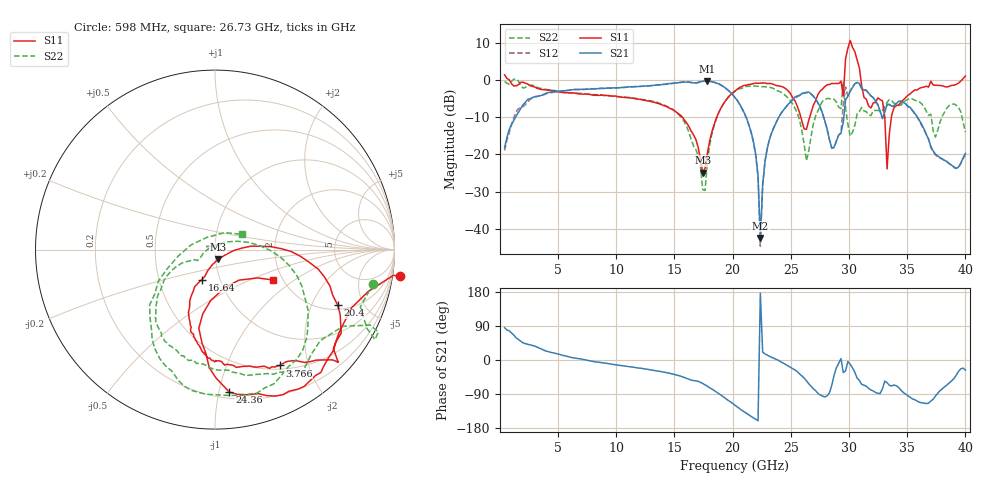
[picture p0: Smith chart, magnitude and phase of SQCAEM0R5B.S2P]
! Network Analyzer HP8722ES.07.66: Jul 25, 2000 Serial No. US39175408
! 26 Oct 2004  08:55:13
! Frequency  S11  S21  S12  S22
# HZ  S  DB R  50
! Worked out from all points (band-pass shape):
!   201 points, 400 MHz to 40 GHz, reference 50 ohm
!   highest |S21| = -0.34 dB at 17.82 GHz (marker M1); lowest = -42.4 dB at 22.38 GHz (marker M2)
!   |S21| within 3 dB of the highest: 4.271 GHz to 19.8 GHz (15.53 GHz wide, 129 % of centre); 30.05 GHz to 31.62 GHz (1.57 GHz wide, 5.09 % of centre)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
!   lowest |S11| = -24.9 dB at 17.43 GHz (marker M3), VSWR 1.12, Z = 51.4 - j5.62 ohm
!   |S11| at or under -10 dB: 15.67 GHz to 18.63 GHz (2.96 GHz wide, 17.3 % of centre); 25.86 GHz to 26.62 GHz (763.7 MHz wide, 2.91 % of centre); 33.07 GHz to 33.64 GHz (570.4 MHz wide, 1.71 % of centre)
!   |S22| runs from -29.7 to 0.2 dB; largest |S21 - S12| = 0.27
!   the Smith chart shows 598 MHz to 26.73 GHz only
!   S11 on the Smith chart (normalised r, x): 598 MHz: -4, -13; 3.766 GHz: 0.55, -1.56; 16.64 GHz: 0.82, -0.28; 20.4 GHz: 2.23, -3.16; 24.36 GHz: 0.25, -1.08; 26.73 GHz: 1.77, -0.69
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4e8  1.35 -5.2  -18.14 85.1  -18.98 88.8  -0.45 0.4
5.98e8  0.37 -8.2  -15.49 79.2  -16.19 78.2  -0.89 -12.1
3.766e9  -2.63 -60.9  -4.01 26.1  -3.85 25.8  -2.49 -67.0
7.132e9  -3.84 -84.4  -2.56 1.5  -2.60 0.5  -3.81 -94.6
1.3666e10  -6.39 -106.3  -1.39 -29.8  -1.37 -29.8  -6.25 -132.7
1.6636e10  -14.77 -113.5  -0.82 -54.4  -0.78 -53.8  -17.79 -154.3
1.7428e10  -24.87 -72.6  -0.40 -62.1  -0.41 -61.9  -29.46 166.1
1.7824e10  -19.82 -3.4  -0.34 -69.2  -0.33 -68.9  -22.11 33.4
2.02e10  -3.06 -21.2  -4.80 -119.6  -4.72 -119.8  -3.03 -43.4
2.0398e10  -2.49 -24.4  -5.50 -123.6  -5.55 -124.0  -2.60 -48.6
2.2378e10  -0.90 -53.6  -42.44 176.3  -44.64 162.7  -1.80 -87.3
2.4358e10  -1.96 -84.2  -8.13 -8.5  -8.15 -8.9  -3.76 -121.0
2.6734e10  -8.82 -27.8  -3.78 -69.1  -3.79 -69.3  -15.27 29.6
2.6932e10  -6.84 -25.7  -4.44 -76.0  -4.41 -76.3  -11.89 14.1
2.8912e10  -0.97 -40.2  -16.42 -20.6  -16.40 -20.9  -5.94 -75.4
2.9506e10  -4.33 30.5  -11.38 -33.5  -6.52 -21.1  -0.46 100.7
3.01e10  10.57 -70.7  -2.98 -11.4  -3.04 -12.0  -15.09 -79.3
3.0496e10  7.58 -91.5  -1.05 -32.3  -1.05 -32.8  -12.27 -64.6
3.0694e10  5.39 65.0  -0.70 -47.7  -0.74 -48.1  -9.15 120.2
3.1486e10  -5.20 -104.8  -2.78 -69.4  -2.83 -70.4  -8.52 -73.2
3.3466e10  -14.33 8.3  -6.56 -66.8  -6.69 -67.7  -5.27 -73.2
4e10  1.02 -43.5  -19.75 -26.6  -20.03 -26.5  -14.08 -18.9
